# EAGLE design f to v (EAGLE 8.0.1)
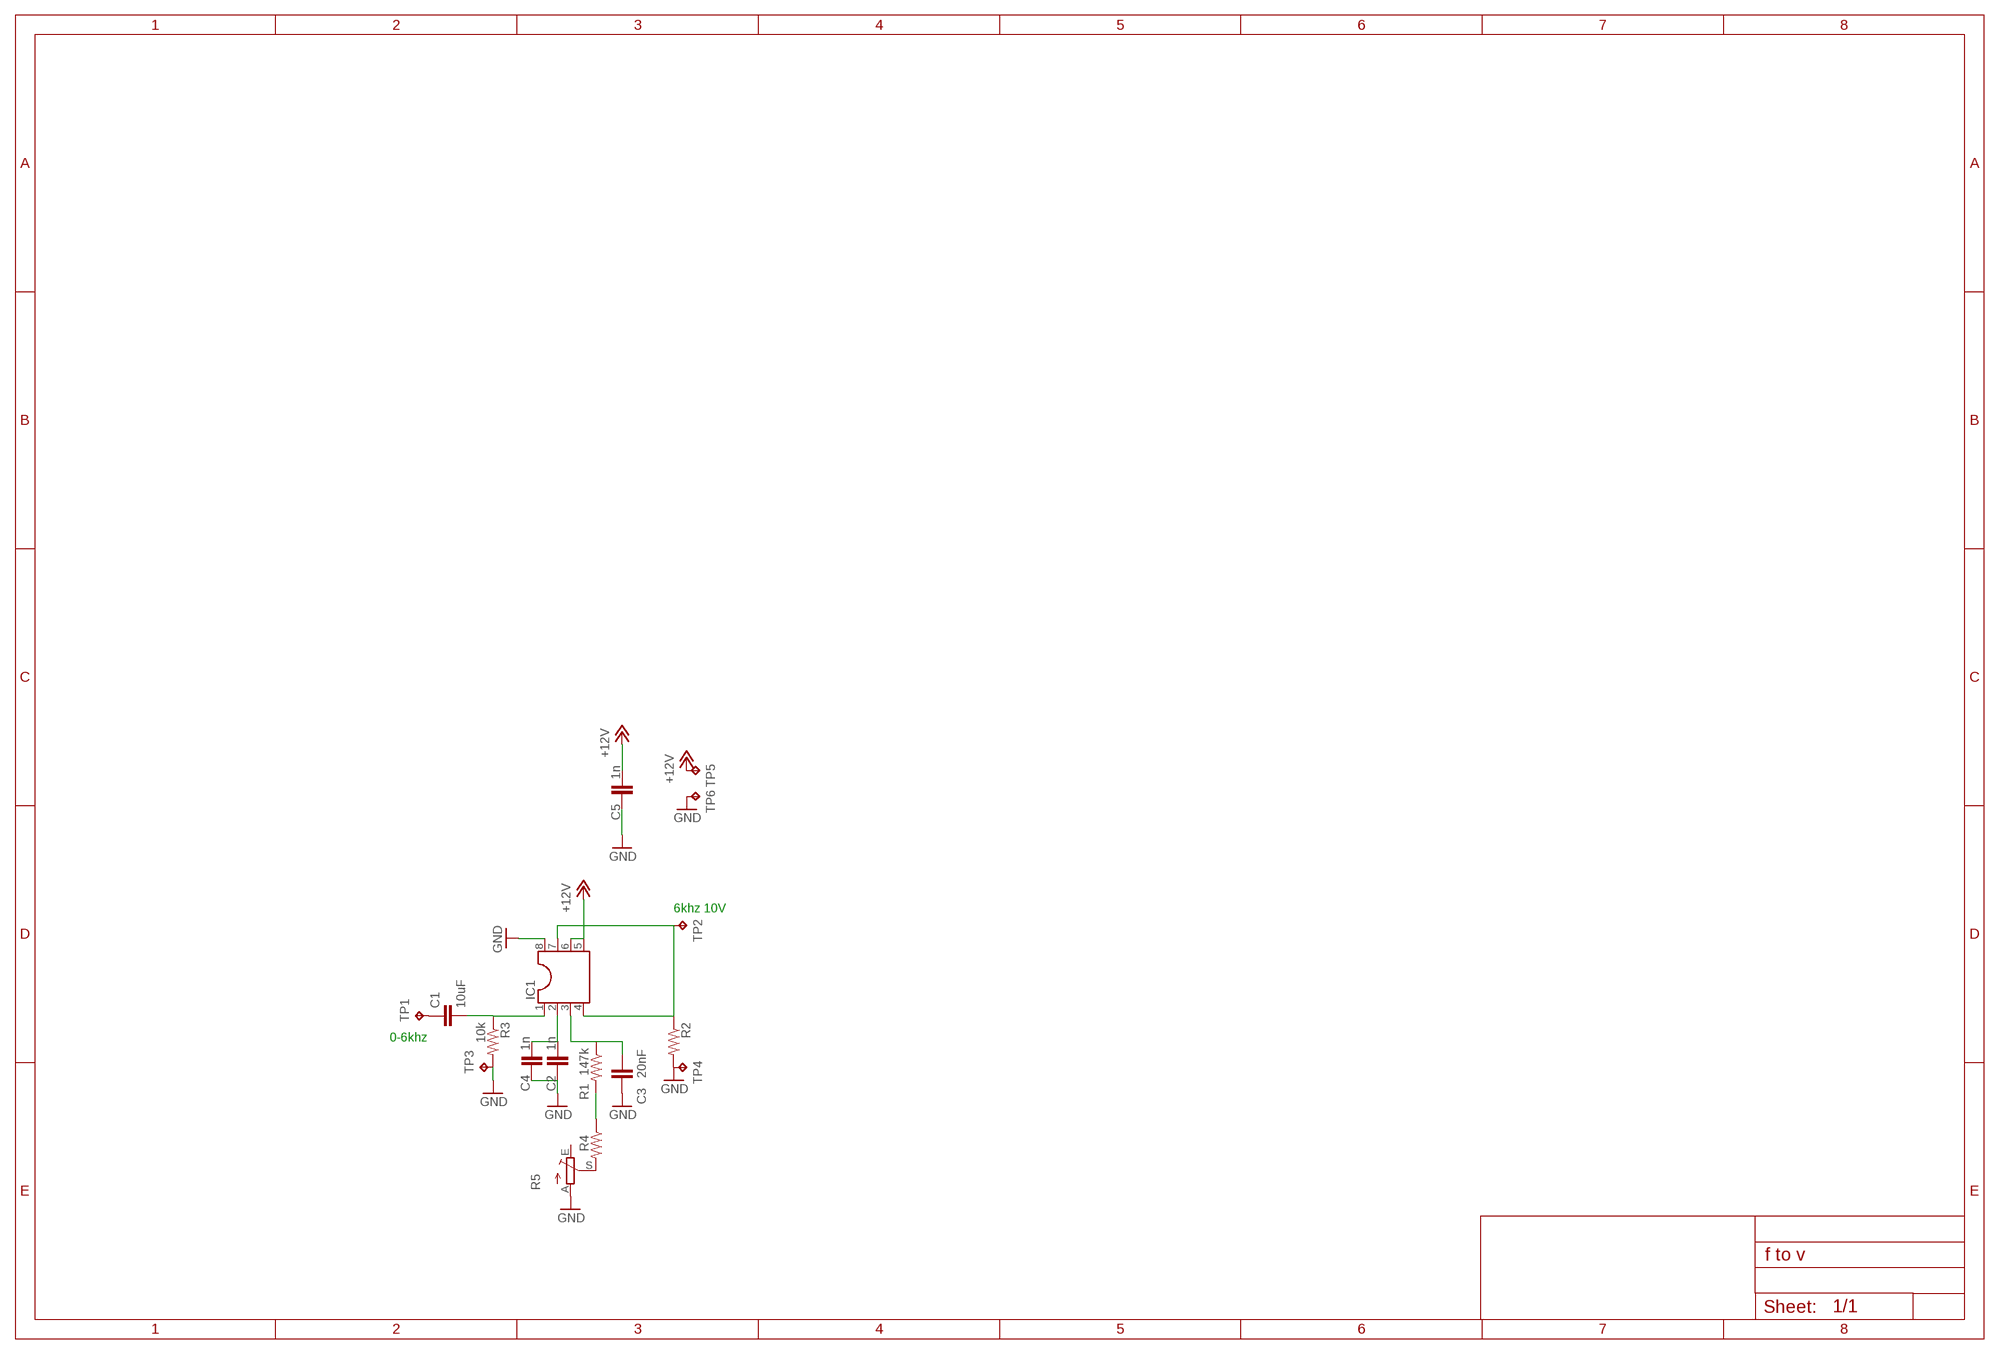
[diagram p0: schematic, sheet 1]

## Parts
C1  10uF  C-EUC0805  [C0805]
C2  1n  C-EUC0805  [C0805]
C3  20nF  C-EUC0805  [C0805]
C4  1n  C-EUC0805  [C0805]
C5  1n  C-EUC0805  [C0805]
IC1  DIL8  [DIL08]
R1  147k  R-US_R0805  [R0805]
R2  R-US_R0805  [R0805]
R3  10k  R-US_R0805  [R0805]
R4  R-US_R0805  [R0805]
R5  TRIM_EU-S64W  [S64W]
TP1  TPPAD1-13  [P1-13]
TP2  TPPAD1-13  [P1-13]
TP3  TPPAD1-13  [P1-13]
TP4  TPPAD1-13  [P1-13]
TP5  TPPAD1-13  [P1-13]
TP6  TPPAD1-13  [P1-13]

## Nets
+12V: C5.2 IC1.5 IC1.6 TP5.TP
GND: C2.1 C3.1 C4.1 C5.1 IC1.8 R2.2 R3.2 R5.A TP3.TP TP4.TP TP6.TP
N$1: R1.2 R4.1
N$2: C1.2 IC1.1 R3.1
N$3: C2.2 C4.2 IC1.2
N$4: C3.2 IC1.3 R1.1
N$5: IC1.4 IC1.7 R2.1 TP2.TP
N$6: R4.2 R5.S
N$7: C1.1 TP1.TP
Unconnected: R5.E

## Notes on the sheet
- 6khz 10V
- 0-6khz

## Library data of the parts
C1-C5 = rcl nhat son:C-EU: CAPACITOR, European symbol
IC1 = ic-package:DIL8: Dual In Line / Socket
R1-R4 = rcl nhat son:R-US_: RESISTOR, American symbol
R5 = pot:TRIM_EU-: POTENTIOMETER
TP1-TP6 = testpad:TP: Test pad

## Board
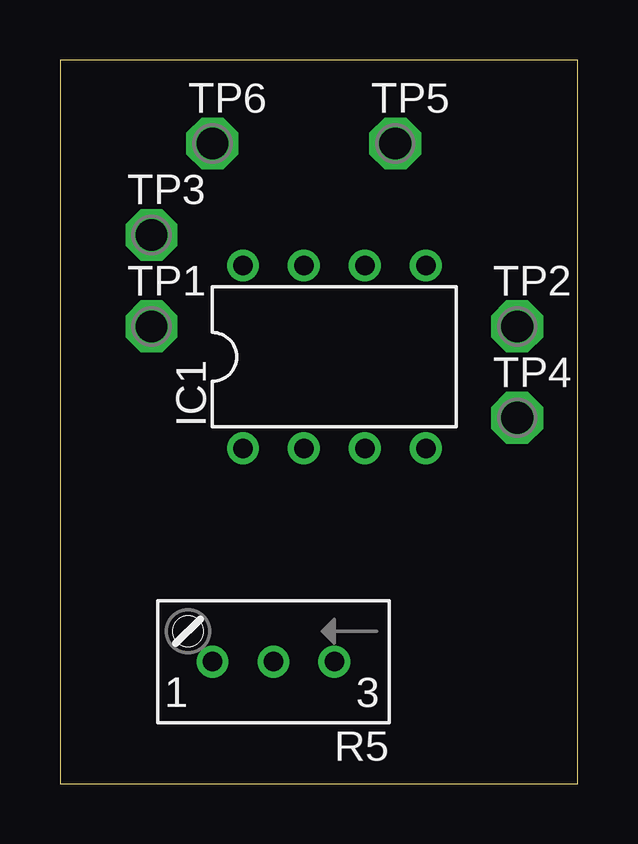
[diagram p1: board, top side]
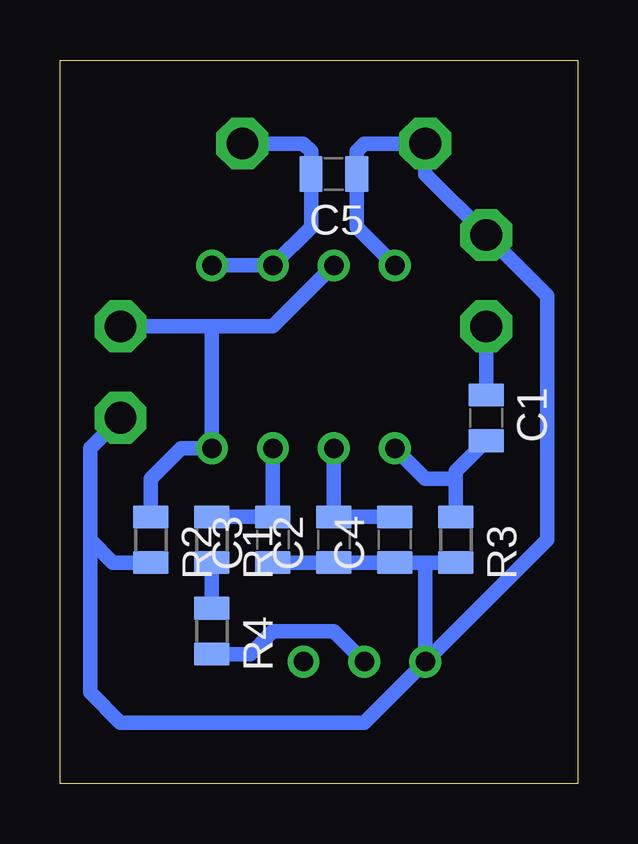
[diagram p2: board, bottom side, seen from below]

Size 21.57 x 30.15 mm. Coordinates in mm from the lower left corner, seen from the top.
Outline: 0,0 21.57,0 21.57,30.15 0,30.15 0,0
Copper layers (1*16): Top 0.035mm / dielectric 1.5mm / Bottom 0.035mm
Design rules "default": minimum track width 10mil, minimum drill 24mil, track to track 8mil, track to pad 8mil, pad to pad 8mil, via to via 8mil, smd to smd 8mil, copper to edge 40mil, drill to drill 8mil, minimum pad ring 10mil, minimum via ring 8mil, stop-mask expansion 4mil, vias tented up to drill 0mil, thermal gap 10mil

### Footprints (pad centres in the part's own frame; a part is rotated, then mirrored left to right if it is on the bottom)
C0805 = smd 0.965 x 1.473: 1 -0.95,0; 2 0.95,0
DIL08 = drill 0.813: 1 -3.81,-3.81; 2 -1.27,-3.81; 3 1.27,-3.81; 4 3.81,-3.81; 5 3.81,3.81; 6 1.27,3.81; 7 -1.27,3.81; 8 -3.81,3.81
R0805 = smd 0.965 x 1.473: 1 -0.95,0; 2 0.95,0
S64W = drill 0.813: A 2.54,1.27; E -2.54,1.27; S 0,1.27
P1-13 = drill 1.321 pad 2.159 octagon: TP 0,0

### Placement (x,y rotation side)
C1  3.81,15.24 270 bottom
C2  10.16,10.16 90 bottom
C3  12.7,10.16 90 bottom
C4  7.62,10.16 90 bottom
C5  10.16,25.4 180 bottom
IC1  11.43,17.78 0 top
R1  15.24,10.16 270 bottom
R2  17.78,10.16 270 bottom
R3  5.08,10.16 270 bottom
R4  15.24,6.35 270 bottom
R5  8.89,6.35 180 top
TP1  3.81,19.05 0 top
TP2  19.05,19.05 0 top
TP3  3.81,22.86 0 top
TP4  19.05,15.24 0 top
TP5  13.97,26.67 0 top
TP6  6.35,26.67 0 top

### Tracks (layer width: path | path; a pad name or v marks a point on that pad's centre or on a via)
+12V
  Bottom 0.61: IC1.5 IC1.6 11.11,23.18 C5.2 11.11,26.35 11.43,26.67 TP5.TP
GND
  Bottom 0.61: IC1.8 9.21,23.18 C5.1 9.21,26.35 8.89,26.67 TP6.TP 6.35,25.4 TP3.TP 1.27,20.32 1.27,10.16 R5.A | TP4.TP 20.32,13.97 20.32,10.16 | R2.2 19.37,9.21 20.32,10.16 | 6.35,9.21 C4.1 C2.1 C3.1 | 6.35,9.21 R3.2 | R5.A 8.89,2.54 19.05,2.54 20.32,3.81 20.32,10.16 | R5.A 6.35,9.21
N$1
  Bottom 0.61: R4.1 R1.2
N$2
  Bottom 0.61: IC1.1 6.35,12.7 5.08,12.7 | 5.08,12.7 R3.1 | C1.2 5.08,13.02 5.08,12.7
N$3
  Bottom 0.61: C4.2 C2.2 IC1.2
N$4
  Bottom 0.61: R1.1 C3.2 IC1.3
N$5
  Bottom 0.61: 15.24,19.05 TP2.TP | 15.24,19.05 12.7,19.05 IC1.7 | 15.24,19.05 IC1.4 16.51,13.97 17.78,12.7 R2.1
N$6
  Bottom 0.61: R4.2 13.65,5.4 12.7,6.35 10.16,6.35 R5.S
N$7
  Bottom 0.61: C1.1 TP1.TP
